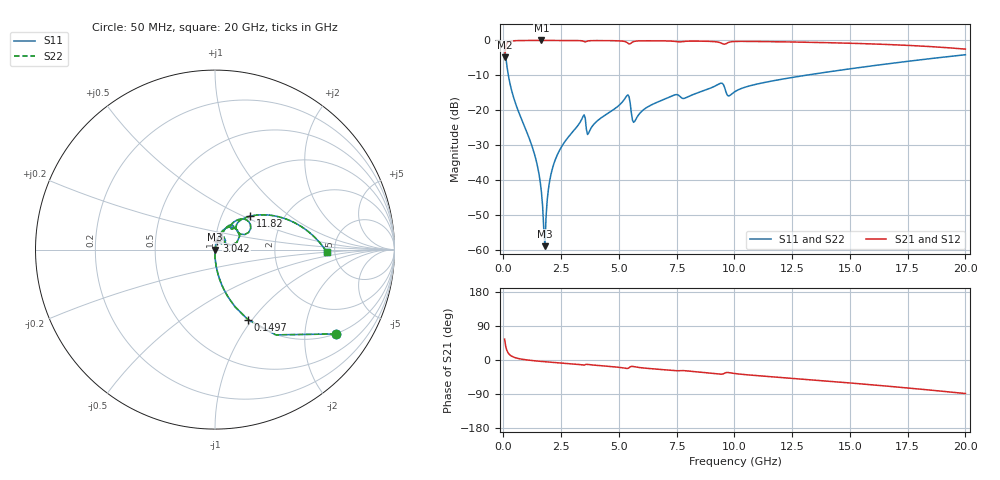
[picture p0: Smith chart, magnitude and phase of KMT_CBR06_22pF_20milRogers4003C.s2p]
! Data measured by Modelithics Inc. support@modelithics.com 813-866-6335
! KEMET CBR0603 22pF, Pad Width= 0.851mm, Pad Length= 0.64mm, Pad Gap= 0.62mm, 20mil Rogers 4003C substrate Data, January 2022
# hz S ma R 50
! 2 Port Network Data from SP1.SP block
! freq  magS11  angS11  magS21  angS21  magS12  angS12  magS22  angS22
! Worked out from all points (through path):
!   401 points, 50 MHz to 20 GHz, reference 50 ohm
!   highest |S21| = -0.01 dB at 1.646 GHz (marker M1); lowest = -4.9 dB at 50 MHz (marker M2)
!   group delay of S21, straight-line fit = 12.7 ps
!   lowest |S11| = -59.0 dB at 1.796 GHz (marker M3), VSWR 1.00, Z = 50.1 + j0.0514 ohm
!   |S11| at or under -10 dB: 213.5 MHz to 13.08 GHz (12.87 GHz wide, 194 % of centre)
!   |S22| runs from -59.0 to -1.7 dB; largest |S21 - S12| = 0
!   S11 on the Smith chart (normalised r, x): 50 MHz: 0.99, -2.87; 149.8 MHz: 0.99, -0.95; 3.042 GHz: 1.02, +0.10; 11.82 GHz: 1.36, +0.54; 20 GHz: 4.30, -0.20
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5e7  0.8207 -35.0  0.5711 55.0  0.5711 55.0  0.8207 -35.0
1.4975e8  0.4303 -64.8  0.9023 25.1  0.9023 25.1  0.4303 -64.8
3.99125e8  0.1688 -81.1  0.9852 8.7  0.9852 8.7  0.1688 -81.1
1.396625e9  0.02015 -90.0  0.9989 -2.4  0.9989 -2.4  0.02015 -90.0
1.646e9  0.006626 -85.9  0.999 -3.8  0.999 -3.8  0.006626 -85.9
1.695875e9  0.004215 -81.4  0.999 -4.1  0.999 -4.1  0.004215 -81.4
1.795625e9  0.001122 27.2  0.999 -4.6  0.999 -4.6  0.001122 27.2
1.995125e9  0.009415 78.2  0.9989 -5.6  0.9989 -5.6  0.009415 78.2
2.194625e9  0.01755 79.9  0.9987 -6.6  0.9987 -6.6  0.01755 79.9
3.0425e9  0.05092 77.2  0.9967 -10.6  0.9967 -10.6  0.05092 77.2
3.391625e9  0.07435 69.9  0.9877 -12.8  0.9877 -12.8  0.07435 69.9
3.690875e9  0.0472 63.5  0.9869 -11.9  0.9869 -11.9  0.0472 63.5
5.33675e9  0.1606 50.1  0.9395 -22.3  0.9395 -22.3  0.1606 50.1
5.685875e9  0.06947 50.1  0.9719 -18.0  0.9719 -18.0  0.06947 50.1
6.73325e9  0.1333 63.4  0.9862 -24.6  0.9862 -24.6  0.1333 63.4
9.376625e9  0.2415 43.0  0.9302 -37.3  0.9302 -37.3  0.2415 43.0
9.72575e9  0.1605 36.0  0.9309 -33.0  0.9309 -33.0  0.1605 36.0
1.0025e10  0.1847 49.2  0.9664 -35.8  0.9664 -35.8  0.1847 49.2
1.18205e10  0.2692 43.6  0.9574 -45.3  0.9574 -45.3  0.2692 43.6
1.336662e10  0.3269 36.4  0.9385 -52.6  0.9385 -52.6  0.3269 36.4
1.670825e10  0.4652 19.0  0.8723 -69.5  0.8723 -69.5  0.4652 19.0
2e10  0.6233 -1.3  0.7506 -88.5  0.7506 -88.5  0.6233 -1.3
